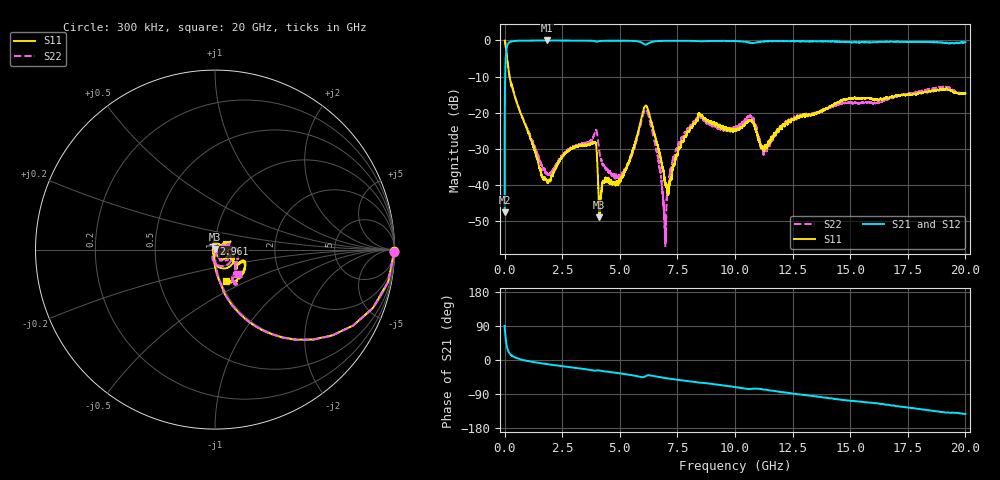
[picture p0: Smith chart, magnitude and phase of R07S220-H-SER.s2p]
!{R07S220}
!Johanson Technology Inc.
!www.johansontechnology.com
!Test Board Conditions:
!Substrate Type  RO4350B
!Substrate Thickness  10 mil
!Substrate Dk  3.66
!TL Type: GCPW
!TL Trace Width  21 mil
!TL Gap  20 mil
!Electrode orientation  Horizontal
!DUT TOPOLOGY	SERIES
!Mounting Pad LxW  16x21 mil
! Created Sat Feb  6 11:50:57 2021
# hz S ma R 50
! 2 Port Network Data from SP1.SP block
! freq  magS11  angS11  magS21  angS21  magS12  angS12  magS22  angS22
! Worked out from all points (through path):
!   20001 points, 300 kHz to 20 GHz, reference 50 ohm
!   highest |S21| = -0.01 dB at 1.833 GHz (marker M1); lowest = -47.6 dB at 300 kHz (marker M2)
!   group delay of S21, straight-line fit = 20.7 ps
!   lowest |S11| = -49.0 dB at 4.113 GHz (marker M3), VSWR 1.01, Z = 50.2 + j0.3 ohm
!   |S11| at or under -10 dB: 215.8 MHz to end of sweep
!   |S22| runs from -57.0 to 0.0 dB; largest |S21 - S12| = 0.013
!   S11 on the Smith chart (normalised r, x): 300 kHz: open; 2.961 GHz: 0.98, +0.06; 20 GHz: 1.06, -0.38
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300000  0.9977 -0.6  0.004177 89.9  0.004238 89.5  1 -0.7
1.023e8  0.5755 -55.5  0.8138 34.8  0.8157 34.6  0.5767 -55.5
1.683e8  0.3932 -68.2  0.9169 22.1  0.9165 22.1  0.3926 -68.4
1.8333e9  0.01154 -165.3  0.9988 -10.8  0.9976 -10.8  0.01453 -40.3
2.9613e9  0.03199 105.2  0.9941 -20.0  0.9952 -19.9  0.03399 26.4
3.3343e9  0.03498 98.3  0.9941 -22.9  0.9947 -22.9  0.03711 27.3
3.9093e9  0.03861 60.6  0.9771 -28.0  0.9765 -28.2  0.0516 21.4
4.1133e9  0.003539 57.6  0.9798 -27.7  0.9808 -27.7  0.02897 -19.6
5.0813e9  0.01329 35.8  0.9913 -36.0  0.9907 -36.0  0.01417 41.7
6.1053e9  0.1243 -37.8  0.8768 -43.4  0.8782 -43.4  0.109 -36.4
6.6673e9  0.03238 -100.4  0.9808 -44.6  0.9818 -44.7  0.02347 -118.0
6.9623e9  0.01081 -74.8  0.9874 -47.6  0.9869 -47.5  0.002101 -44.2
7.1363e9  0.009381 -11.6  0.9888 -49.0  0.9872 -49.0  0.01085 24.4
7.3723e9  0.01899 26.0  0.9878 -51.0  0.9878 -51.0  0.02436 29.7
8.1263e9  0.06259 33.6  0.9846 -57.1  0.9844 -57.1  0.06674 22.0
8.4873e9  0.09343 27.6  0.9755 -59.8  0.9752 -59.8  0.0872 21.6
1.00003e10  0.05839 27.1  0.9792 -71.5  0.9801 -71.5  0.05833 -9.2
1.07263e10  0.07766 -38.6  0.9231 -76.2  0.9215 -76.1  0.08596 -44.1
1.13033e10  0.03432 -38.5  0.9713 -78.2  0.9712 -78.3  0.03245 -24.8
1.33343e10  0.09451 -27.9  0.9716 -94.6  0.9731 -94.7  0.09633 6.5
1.66673e10  0.1588 -24.6  0.9541 -118.4  0.9598 -118.7  0.1561 -41.9
2e10  0.1852 -70.1  0.946 -142.7  0.9386 -142.6  0.1883 -47.5
